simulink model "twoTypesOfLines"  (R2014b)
settings: Solver=ode45  StartTime=0.0  StopTime=1000  RelTol=1e-3

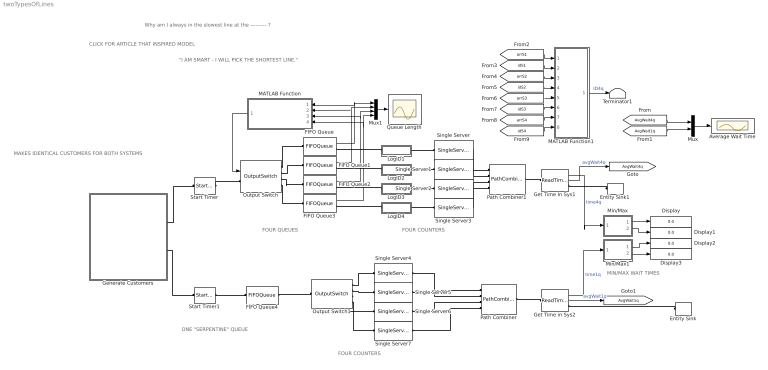
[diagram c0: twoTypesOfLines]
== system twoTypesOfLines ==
  note: Why am I always in the slowest line at the --------- ?
  note: MAKES IDENTICAL CUSTOMERS FOR BOTH SYSTEMS
  note: "I AM SMART - I WILL PICK THE SHORTEST LINE."
  note: ONE "SERPENTINE" QUEUE
  note: FOUR COUNTERS
  note: FOUR COUNTERS
  note: FOUR QUEUES
  note: CLICK FOR ARTICLE THAT INSPIRED MODEL
  note: MIN/MAX WAIT TIMES
  Average Wait Time : Scope
  Display{,1..3} (4 alike) : Display
  Entity Sink : EntitySink
  Entity Sink1 : EntitySink
  FIFO Queue{,1..3} (4 alike) : FIFOQueue  Capacity=inf  StatNumberInBlock=on
  FIFO Queue4 : FIFOQueue  Capacity=inf
  Generate Customers : Subsystem
  Get Time In Sys1 : ReadTimer  StatTimeElapsed=on  StatAverageTimeElapsed=on
  Get Time in Sys2 : ReadTimer  TimerTag=T2  StatTimeElapsed=on  StatAverageTimeElapsed=on
  LogID1 : Subsystem
  LogID2 : Subsystem
  LogID3 : Subsystem
  LogID4 : Subsystem
  MATLAB Function : MATLAB Function  TreatAsAtomicUnit=on
  MATLAB Function1 : MATLAB Function  TreatAsAtomicUnit=on
  Min/Max : Subsystem  TreatAsAtomicUnit=on
  Min/Max1 : Subsystem  TreatAsAtomicUnit=on
  Mux : Mux  Inputs=2
  Mux1 : Mux
  Output Switch : OutputSwitch  NumberOutputPorts=4  SwitchingCriterion=From signal port p  InitialConditionsOpt=on
  Output Switch1 : OutputSwitch  NumberOutputPorts=4
  Path Combiner : PathCombiner  NumberInputPorts=4
  Path Combiner1 : PathCombiner  NumberInputPorts=4
  Queue Length : Scope
  Single Server{,1..7} (8 alike) : SingleServer  ServiceTimeFrom=Attribute  AttributeName=sTime
  Start Timer : StartTimer
  Start Timer1 : StartTimer  TimerTag=T2
  Terminator1 : Terminator
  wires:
  FIFO Queue/1 -> MATLAB Function/1(n1), Mux1/1
  FIFO Queue1/1 -> Mux1/2, MATLAB Function/2(n2)
  FIFO Queue2/1 -> Mux1/3, MATLAB Function/3(n3)
  FIFO Queue3/1 -> Mux1/4, MATLAB Function/4(n4)
  MATLAB Function/1(sq) -> Output Switch/1
  Mux/1 -> Average Wait Time/1
  Mux1/1 -> Queue Length/1
  Get Time In Sys1/1 -> Min/Max/1(u)  "time4q"
  Get Time in Sys2/1 -> Min/Max1/1(u)  "time1q"
  Min/Max/1(min) -> Display/1
  Min/Max/2(max) -> Display1/1
  Min/Max1/1(min) -> Display2/1
  Min/Max1/2(max) -> Display3/1
  Get Time In Sys1/2 -> [AvgWait4q]  "avgWait4q"
  Get Time in Sys2/2 -> [AvgWait1q]  "avgWait1q"
  [AvgWait4q] -> Mux/1
  [AvgWait1q] -> Mux/2
  [idS3] -> MATLAB Function1/6(id3)
  [idS4] -> MATLAB Function1/8(id4)
  [arrS3] -> MATLAB Function1/5(arr3)
  [idS1] -> MATLAB Function1/2(id1)
  [arrS1] -> MATLAB Function1/1(arr1)
  [arrS4] -> MATLAB Function1/7(arr4)
  [idS2] -> MATLAB Function1/4(id2)
  [arrS2] -> MATLAB Function1/3(arr2)
  MATLAB Function1/1(id) -> Terminator1/1  "ID4q"
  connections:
  Output Switch/RConn1 -- FIFO Queue/LConn1
  Output Switch/RConn2 -- FIFO Queue1/LConn1
  Output Switch/RConn3 -- FIFO Queue2/LConn1
  Output Switch/RConn4 -- FIFO Queue3/LConn1
  Start Timer1/RConn1 -- FIFO Queue4/LConn1
  LogID2/LConn1 -- FIFO Queue1/RConn1
  LogID3/LConn1 -- FIFO Queue2/RConn1
  LogID4/LConn1 -- FIFO Queue3/RConn1
  Output Switch1/RConn1 -- Single Server4/LConn1
  Output Switch1/RConn2 -- Single Server5/LConn1
  Output Switch1/RConn3 -- Single Server6/LConn1
  Output Switch1/RConn4 -- Single Server7/LConn1
  FIFO Queue4/RConn1 -- Output Switch1/LConn1
  Single Server4/RConn1 -- Path Combiner/LConn1
  Single Server5/RConn1 -- Path Combiner/LConn2
  Single Server6/RConn1 -- Path Combiner/LConn3
  Single Server7/RConn1 -- Path Combiner/LConn4
  Entity Sink/LConn1 -- Get Time in Sys2/RConn1
  Single Server/RConn1 -- Path Combiner1/LConn1
  Single Server1/RConn1 -- Path Combiner1/LConn2
  Single Server2/RConn1 -- Path Combiner1/LConn3
  Single Server3/RConn1 -- Path Combiner1/LConn4
  Start Timer/RConn1 -- Output Switch/LConn1
  Get Time In Sys1/LConn1 -- Path Combiner1/RConn1
  Get Time in Sys2/LConn1 -- Path Combiner/RConn1
  Entity Sink1/LConn1 -- Get Time In Sys1/RConn1
  Generate Customers/RConn1 -- Start Timer/LConn1
  Generate Customers/RConn2 -- Start Timer1/LConn1
  LogID1/LConn1 -- FIFO Queue/RConn1
  Single Server/LConn1 -- LogID1/RConn1
  Single Server1/LConn1 -- LogID2/RConn1
  Single Server2/LConn1 -- LogID3/RConn1
  Single Server3/LConn1 -- LogID4/RConn1

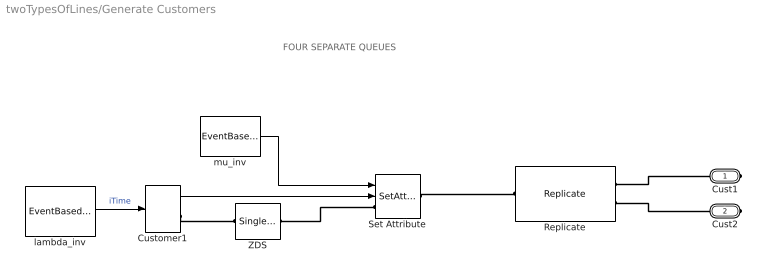
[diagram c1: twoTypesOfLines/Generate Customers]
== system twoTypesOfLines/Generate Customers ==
  note: FOUR SEPARATE QUEUES
  Customer1 : TimeBasedEntityGenerator  GenerateEntitiesUpon=Intergeneration time from port t  Distribution=Exponential  InitialSeed=35250  Mean=0.9  GenerateEntityAtSimulationStart=off  StatNumberDeparted=on
  Replicate : Replicate  NumberOutputPorts=2
  Set Attribute : SetAttribute  AttributeName=sTime|ID  AttributeFrom=Signal port|Signal port  AttributeValue=1|1  AttributeTreatAsVector=1|1  EvaluatedAttributeValue={ [];[]}
  ZDS : SingleServer  ServiceTime=0  AttributeName=sTime
  lambda_inv : EventBasedRandomNumber  Seed=35250
  mu_inv : EventBasedRandomNumber  meanExp=2  Seed=30384
  Cust1 : PMIOPort  Port=1  Side=Right
  Cust2 : PMIOPort  Port=2  Side=Right
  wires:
  mu_inv/1 -> Set Attribute/1
  Customer1/1 -> Set Attribute/2
  lambda_inv/1 -> Customer1/1  "iTime"
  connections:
  Replicate/RConn1 -- Cust1/RConn1
  Customer1/RConn1 -- ZDS/LConn1
  Replicate/RConn2 -- Cust2/RConn1
  ZDS/RConn1 -- Set Attribute/LConn1
  Set Attribute/RConn1 -- Replicate/LConn1

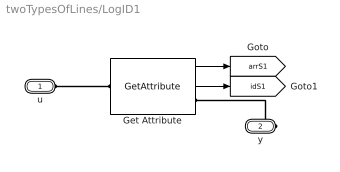
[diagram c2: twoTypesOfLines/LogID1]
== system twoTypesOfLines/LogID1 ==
  Get Attribute : GetAttribute  AttributeName=ID  StatNumberDeparted=on  EvaluatedDefaultAttributeValue={ []}
  u : PMIOPort  Port=1  Side=Left
  y : PMIOPort  Port=2  Side=Right
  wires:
  Get Attribute/1 -> [arrS1]
  Get Attribute/2 -> [idS1]
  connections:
  y/RConn1 -- Get Attribute/RConn1
  Get Attribute/LConn1 -- u/RConn1

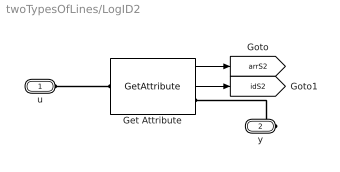
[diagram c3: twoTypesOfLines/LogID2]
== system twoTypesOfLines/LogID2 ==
  Get Attribute : GetAttribute  AttributeName=ID  StatNumberDeparted=on  EvaluatedDefaultAttributeValue={ []}
  u : PMIOPort  Port=1  Side=Left
  y : PMIOPort  Port=2  Side=Right
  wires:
  Get Attribute/1 -> [arrS2]
  Get Attribute/2 -> [idS2]
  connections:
  y/RConn1 -- Get Attribute/RConn1
  Get Attribute/LConn1 -- u/RConn1

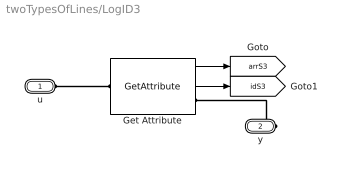
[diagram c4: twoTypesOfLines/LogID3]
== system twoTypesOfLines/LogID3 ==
  Get Attribute : GetAttribute  AttributeName=ID  StatNumberDeparted=on  EvaluatedDefaultAttributeValue={ []}
  u : PMIOPort  Port=1  Side=Left
  y : PMIOPort  Port=2  Side=Right
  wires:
  Get Attribute/1 -> [arrS3]
  Get Attribute/2 -> [idS3]
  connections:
  y/RConn1 -- Get Attribute/RConn1
  Get Attribute/LConn1 -- u/RConn1

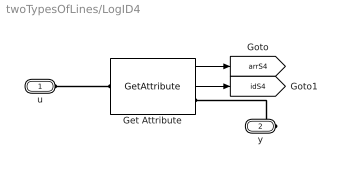
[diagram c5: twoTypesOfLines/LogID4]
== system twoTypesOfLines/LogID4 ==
  Get Attribute : GetAttribute  AttributeName=ID  StatNumberDeparted=on  EvaluatedDefaultAttributeValue={ []}
  u : PMIOPort  Port=1  Side=Left
  y : PMIOPort  Port=2  Side=Right
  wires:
  Get Attribute/1 -> [arrS4]
  Get Attribute/2 -> [idS4]
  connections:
  y/RConn1 -- Get Attribute/RConn1
  Get Attribute/LConn1 -- u/RConn1

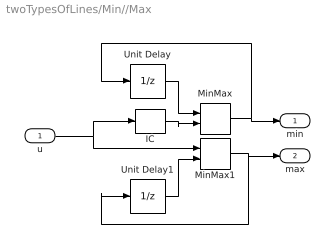
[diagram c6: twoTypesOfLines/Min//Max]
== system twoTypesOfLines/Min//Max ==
  u : Inport
  IC : InitialCondition  Value=100
  MinMax : MinMax  Inputs=2
  MinMax1 : MinMax  Function=max  Inputs=2
  Unit Delay : UnitDelay  InitialCondition=100  SampleTime=-1
  Unit Delay1 : UnitDelay  SampleTime=-1
  min : Outport
  max : Outport  Port=2
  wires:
  Unit Delay1/1 -> MinMax1/2
  MinMax1/1 -> Unit Delay1/1, max/1
  Unit Delay/1 -> MinMax/1
  MinMax/1 -> Unit Delay/1, min/1
  u/1 -> MinMax1/1, IC/1
  IC/1 -> MinMax/2

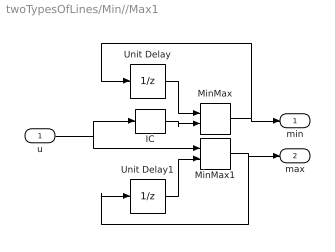
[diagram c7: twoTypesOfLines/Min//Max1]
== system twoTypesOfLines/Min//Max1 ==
  u : Inport
  IC : InitialCondition  Value=100
  MinMax : MinMax  Inputs=2
  MinMax1 : MinMax  Function=max  Inputs=2
  Unit Delay : UnitDelay  InitialCondition=100  SampleTime=-1
  Unit Delay1 : UnitDelay  SampleTime=-1
  min : Outport
  max : Outport  Port=2
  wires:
  IC/1 -> MinMax/2
  u/1 -> IC/1, MinMax1/1
  MinMax/1 -> min/1, Unit Delay/1
  Unit Delay/1 -> MinMax/1
  MinMax1/1 -> max/1, Unit Delay1/1
  Unit Delay1/1 -> MinMax1/2

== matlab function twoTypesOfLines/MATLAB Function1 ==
function id = idMerge(arr1,id1,arr2,id2,arr3,id3,arr4,id4)
%#codegen
persistent arr1S arr2S arr3S arr4S

if isempty(arr1S)
    arr1S = 1;
end
if isempty(arr2S)
    arr2S = 1;
end
if isempty(arr3S)
    arr3S = 1;
end
if isempty(arr4S)
    arr4S = 1;
end
id = 0;
if arr1 ~= arr1S
    id = id1;
    arr1S = arr1;
elseif arr2 ~= arr2S
    id = id2;
    arr2S = arr2;
elseif arr3 ~= arr3S
    id = id3;
    arr3S = arr3;
elseif arr4 ~= arr4S
    id = id4;
    arr4S = arr4;
end

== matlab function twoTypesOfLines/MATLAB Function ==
function sq = shortestQueue(n1,n2,n3,n4)
%#codegen

% Pick a short queue at random
nVals = [n1, n2, n3, n4];
minVal = min(nVals);
minIdx = find(nVals == minVal);
randSel = randi([1 length(minIdx)]);
sq = minIdx(randSel);
